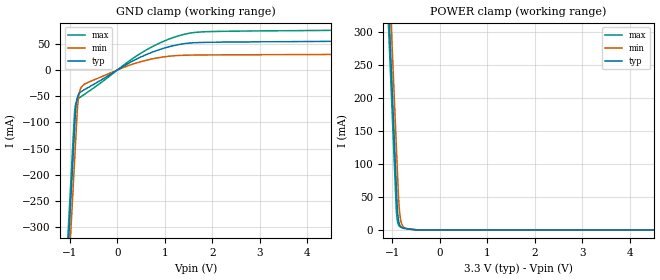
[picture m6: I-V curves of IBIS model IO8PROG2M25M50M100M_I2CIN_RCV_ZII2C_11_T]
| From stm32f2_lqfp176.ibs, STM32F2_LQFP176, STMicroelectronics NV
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| *** New cell (Generated with 5.14beta1 (Sep 20 2010 13:23:23))
[Model]   IO8PROG2M25M50M100M_I2CIN_RCV_ZII2C_11_T
Model_type Input
Polarity   Non-Inverting
Enable   Active-Low
| CAP_THRESHOLD on pad IOV33 is "CMOS" :
| Rising=10.0% of vddio   Falling=90.0% of vddio
| C_comp min and max val. don't necessarily correlate with the min and max pvt
| but are the smallest and greatest pad capacitance found.
| var   typ   min   max
C_comp   2.13955pF  2.03575pF  2.25660pF
Vinl = 800.0mV | Dummy value overriden by next lines
Vinh = 2.00V | Dummy value overriden by next lines
[Model Spec]
| TIME_THRESHOLD on pin ZII2CV12 is "CORE" :
| Rising=40.0% of vdd   Falling=60.0% of vdd
Vinl 1.25450V 1.03850V 1.36250V
Vinh 1.66150V 1.36950V 1.82450V
| variable   typ   min   max
[Temperature Range] 25.0 125.0 -40.0
| variable   typ   min   max
[Voltage Range] 3.3V 2.7V 3.6V
| variable   typ   min   max
[POWER Clamp Reference] 3.3V 2.7V 3.6V
| variable   typ   min   max
[GND Clamp Reference] 0V 0V 0V
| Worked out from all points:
|   GND clamp passes 1 mA (typ) near -0.02 V on its own axis
|   POWER clamp passes 1 mA (typ) near -0.62 V on its own axis
[POWER Clamp]
-3.3V     4.113A     4.176A     4.076A
-1.09V    357mA      419.2mA    320.8mA
-1.05V    289mA      351.2mA    252.8mA
-1.01V    221mA      283.2mA    184.9mA
-920mV    68.07mA    130.3mA    32.01mA
-910mV    51.08mA    113.3mA    21.64mA
-890mV    25.6mA     79.28mA    11.28mA
-860mV    10.4mA     36.05mA    6.133mA
-830mV    5.371mA    16.57mA    4.527mA
-790mV    3.177mA    6.724mA    3.572mA
-340mV    0A         46uA       21uA
6.6V      0A         0A         0A
[GND Clamp]
-3.3V     -4.189A    -4.249A    -4.155A
-1.06V    -380.8mA   -441.1mA   -346.5mA
-940mV    -176.8mA   -237.1mA   -142.5mA
-900mV    -108.8mA   -169.1mA   -78.46mA
-870mV    -66.81mA   -118.1mA   -61.62mA
-840mV    -51.26mA   -70.71mA   -56.41mA
-810mV    -45.36mA   -47.08mA   -53.83mA
-770mV    -41.78mA   -34.45mA   -51.23mA
120mV     6.714mA    4.461mA    8.567mA
950mV     40.72mA    24.58mA    53.81mA
1.77V     52.39mA    28.47mA    72.51mA
6.6V      55.76mA    30.09mA    76.94mA
